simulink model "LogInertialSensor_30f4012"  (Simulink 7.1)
settings: Solver=FixedStepDiscrete  StartTime=0.0  StopTime=10.0  FixedStep=0.001  RelTol=1e-3
undefined symbols (not defined in the file or in its folder): bin2dec, bits, Buffer, characters, contain, empty, has, hex2dec, one, space, Transmit, When
libraries: dsPICdrivers x41, simulink x25

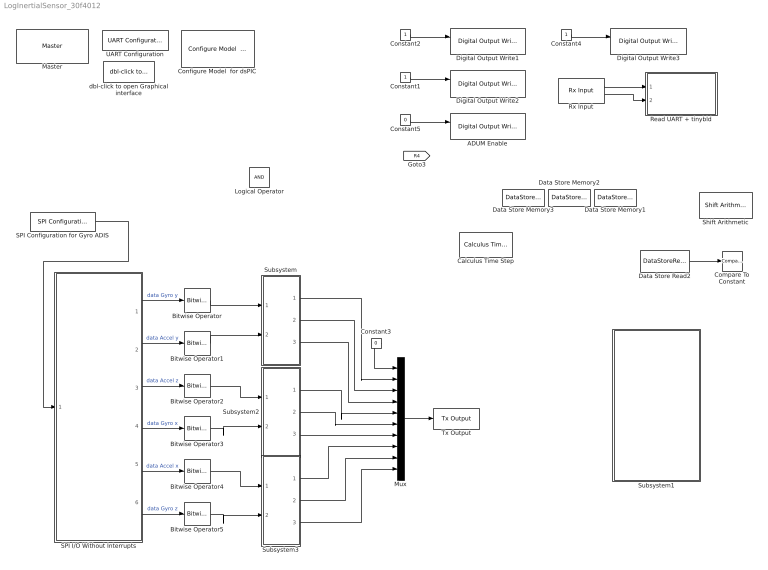
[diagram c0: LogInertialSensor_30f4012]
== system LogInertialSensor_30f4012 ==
  ADUM Enable : dsPICdrivers/Digital I//O/Digital Output Write  Tag=dsPIC_Digital_Output  Priority=5  PORT=E  Pin=1  Simultaneous=off  OrderingInOutPopup=Input
  Bitwise Operator{,1..5} (6 alike) : simulink/Logic and Bit Operations/Bitwise Operator  logicop=AND  UseBitMask=on  BitMask=hex2dec('0FFF')  BitMaskRealWorld=Stored Integer
  Calculus Time Step : dsPICdrivers/OTHERS/Calculus Time Step  Tag=dsPIC_CalculusTimeStep  SampleTime=.001  PR1chk=on
  Compare To Constant : simulink/Logic and Bit Operations/Compare To Constant  SystemSampleTime=-1  relop===  const=1  LogicOutDataTypeMode=uint8  ZeroCross=off
  Configure Model  for dsPIC : dsPICdrivers/Simulink Configuration/Configure Model  for dsPIC
  Constant1 : Constant  OutDataTypeMode=boolean  OutDataType=sfix(16)  OutScaling=2^0  OutDataTypeStr=boolean  SampleTime=-1
  Constant2 : Constant  OutDataTypeMode=boolean  OutDataType=sfix(16)  OutScaling=2^0  OutDataTypeStr=boolean  SampleTime=-1
  Constant3 : Constant  Value=0  OutDataTypeMode=uint8  OutDataType=sfix(16)  OutScaling=2^0  OutDataTypeStr=uint8  SampleTime=-1
  Constant4 : Constant  OutDataTypeMode=boolean  OutDataType=sfix(16)  OutScaling=2^0  OutDataTypeStr=boolean  SampleTime=-1
  Constant5 : Constant  Value=0  OutDataTypeMode=boolean  OutDataType=sfix(16)  OutScaling=2^0  OutDataTypeStr=boolean  SampleTime=-1
  Data Store Memory1 : DataStoreMemory  DataStoreName=Variable62  ReadBeforeWriteMsg=warning  WriteAfterWriteMsg=warning  WriteAfterReadMsg=warning  DataType=uint8  OutDataType=sfix(16)  OutScaling=2^0  OutDataTypeStr=uint8
  Data Store Memory2 : DataStoreMemory  DataStoreName=Variable61  ReadBeforeWriteMsg=warning  WriteAfterWriteMsg=warning  WriteAfterReadMsg=warning  DataType=uint8  OutDataType=sfix(16)  OutScaling=2^0  OutDataTypeStr=uint8
  Data Store Memory3 : DataStoreMemory  DataStoreName=Variable60  ReadBeforeWriteMsg=warning  WriteAfterWriteMsg=warning  WriteAfterReadMsg=warning  DataType=uint8  OutDataType=sfix(16)  OutScaling=2^0  OutDataTypeStr=uint8
  Data Store Read2 : DataStoreRead  DataStoreName=Variable60  SampleTime=.01
  Digital Output Write1 : dsPICdrivers/Digital I//O/Digital Output Write  Tag=dsPIC_Digital_Output  Priority=5  PORT=E  Pin=5  Simultaneous=off  OrderingInOutPopup=Input & Output
  Digital Output Write2 : dsPICdrivers/Digital I//O/Digital Output Write  Tag=dsPIC_Digital_Output  Priority=5  PORT=E  Pin=3  Simultaneous=off  OrderingInOutPopup=Input & Output
  Digital Output Write3 : dsPICdrivers/Digital I//O/Digital Output Write  Tag=dsPIC_Digital_Output  Priority=5  PORT=B  Pin=0  Simultaneous=off  OrderingInOutPopup=Input & Output
  Logical Operator : Logic  AllPortsSameDT=off  OutDataTypeMode=boolean  OutDataTypeStr=boolean
  Master : dsPICdrivers/Master  Tag=dsPIC_MASTER  Priority=1  TimeStepType=Timer1  picType=30f4012  fcy=20e6  Quartz_33f=5e6  PLLActive_33f=off  fcyDesired_33f=0  tmr1="[1  19999  0]"  tmr1Info="Time Step : 0.001  ;   Error : 0%  PR1=19999"  tmr2345="[0  0  0  0]"  tmr2345cfg=[-1 -1 -1 -1]  IOautoConf=on  typePort="[ 0   0   0   0   0   0   0   0   0   0   0   0   0   0   0   0  10   0   0   0   0   0   0   0   0   0   0   0   0   0   0   0   0   0   0   0   0   0   0   0   0   0   0   0   0   5   4   0   0   0   0   0   0   0   0   0   0   0   0   0   0   0   0   0   0  10   0  10   0  10   0   0  17   0   0   0   0   0   0   0   0   0  14  15   0   0   0   0   0   0   0   0   0   0   0   0   0   0   0   0 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"  TRIS="[ 65535  65534  65535  65535  65493  65535  65535 ]"  ADPCFG=1  MasterBusyPort=None  MasterOverloadPort=None  FOSC=XT_PLL8  ClockSwitchMonitor=Both disabled  TempProtection_33f=TEMP_ON  FPBOR=PBOR_OFF  PWRT=PWRT_4  MCLR=MCLR_DIS  PowerSave=off  OverrideFcy=off  NewFcy=1e6
  Mux : Mux  Inputs=10
  Read UART + tinybld : Subsystem  TreatAsAtomicUnit=on
  Rx Input : dsPICdrivers/Serial PORT/Rx Input  Tag=dsPIC_RX  Priority=5  UART=1  SampleTime=.01  BlockingFctChk=off  OutputDefault=0  IsPresentFlagChk=on
  SPI Configuration for Gyro ADIS : dsPICdrivers/SPI PORT/SPI Configuration  Tag=dsPIC_config_SPI  Priority=2  ConfigurationTime=At block execution (reconfigure on the fly)  OrderingInOutPopup=Output  SampleTime=-1  Frame_Enable=0  Frame_Sync=0  SPI=1  MODE=MASTER  USER_SCALER=2  StartEnable=Enable  SDO_EN=on  DATA_LENGTH=16 bits  SS_EN=off  SMP=Middle of bit  CKP=high  CKE=Idle to Active  Status="OK - Mode 1  -    Fsck= 10000000Hz"
  SPI I/O Without Interrupts : Subsystem
  Shift Arithmetic : simulink/Logic and Bit Operations/Shift Arithmetic  SystemSampleTime=-1  nBitShiftRight=8  nBinPtShiftRight=0
  Subsystem : Subsystem
  Subsystem1 : Subsystem
  Subsystem2 : Subsystem
  Subsystem3 : Subsystem
  Tx Output : dsPICdrivers/Serial PORT/Tx Output  Tag=dsPIC_TX  Priority=5  UART=1  OrderingInOutPopup=None
  UART Configuration : dsPICdrivers/Serial PORT/UART Configuration  Tag=dsPIC_config_UART  Priority=2  UART=1  proposed_BAUD=115200  ALT_TX_RX=on  InterruptTxWhen=When Transmit Buffer has one empty space (contain 3 characters)  TXInterruptPri=4  TxBufferSize=128  TXEN=on  InterruptRxWhen=When a character is received  RXInterruptPri=1  RxBufferSize=32  BAUD=115200  UxBRG=10  Info="UxBRG = 10   ||  Real Baud : 113636   ||  % error : -1.3573  ||  max 11.3636 Bytes / Step"  RealBaud=0
  dbl-click to open Graphical interface : dsPICdrivers/Serial PORT/dbl-click to open Graphical interface  SystemSampleTime=-1  Nothing=0
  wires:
  Constant2/1 -> Digital Output Write1/1
  Constant1/1 -> Digital Output Write2/1
  Constant5/1 -> ADUM Enable/1
  Rx Input/1 -> Read UART + tinybld/1(Rx)
  Rx Input/2 -> Read UART + tinybld/2(Flag)
  Constant4/1 -> Digital Output Write3/1
  SPI Configuration for Gyro ADIS/1 -> SPI I/O Without Interrupts/1(Ordering)
  SPI I/O Without Interrupts/1(Gyro y) -> Bitwise Operator/1  "data Gyro y"
  SPI I/O Without Interrupts/2(Accel y) -> Bitwise Operator1/1  "data Accel y"
  SPI I/O Without Interrupts/3(Accel z) -> Bitwise Operator2/1  "data Accel z"
  SPI I/O Without Interrupts/4(Gyro x) -> Bitwise Operator3/1  "data Gyro x"
  SPI I/O Without Interrupts/5(Accel x) -> Bitwise Operator4/1  "data Accel x"
  SPI I/O Without Interrupts/6(Gyro z) -> Bitwise Operator5/1  "data Gyro z"
  Data Store Read2/1 -> Compare To Constant/1
  Bitwise Operator/1 -> Subsystem/1(In1)
  Bitwise Operator1/1 -> Subsystem/2(In2)
  Bitwise Operator2/1 -> Subsystem2/1(In1)
  Bitwise Operator3/1 -> Subsystem2/2(In2)
  Bitwise Operator4/1 -> Subsystem3/1(In1)
  Bitwise Operator5/1 -> Subsystem3/2(In2)
  Mux/1 -> Tx Output/1
  Constant3/1 -> Mux/1
  Subsystem/1(Out1) -> Mux/2
  Subsystem/2(Out2) -> Mux/3
  Subsystem/3(Out3) -> Mux/4
  Subsystem2/1(Out1) -> Mux/5
  Subsystem2/2(Out2) -> Mux/6
  Subsystem2/3(Out3) -> Mux/7
  Subsystem3/1(Out1) -> Mux/8
  Subsystem3/2(Out2) -> Mux/9
  Subsystem3/3(Out3) -> Mux/10

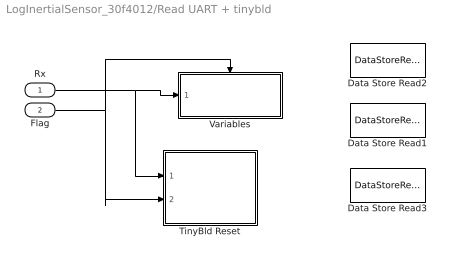
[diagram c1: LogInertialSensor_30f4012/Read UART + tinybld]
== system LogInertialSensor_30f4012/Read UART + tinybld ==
  Rx : Inport  OutDataType=sfix(16)  OutScaling=2^0
  Flag : Inport  Port=2  OutDataType=sfix(16)  OutScaling=2^0
  Data Store Read1 : DataStoreRead  DataStoreName=Variable61  SampleTime=.01
  Data Store Read2 : DataStoreRead  DataStoreName=Variable60  SampleTime=.01
  Data Store Read3 : DataStoreRead  DataStoreName=Variable62  SampleTime=.01
  TinyBld Reset : Subsystem  AncestorBlock=dsPICdrivers/OTHERS/TinyBld Reset
  Variables : Subsystem  TreatAsAtomicUnit=on
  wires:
  Flag/1 -> Variables/Enable, TinyBld Reset/2(Flag)
  Rx/1 -> Variables/1(In1), TinyBld Reset/1(Rx)

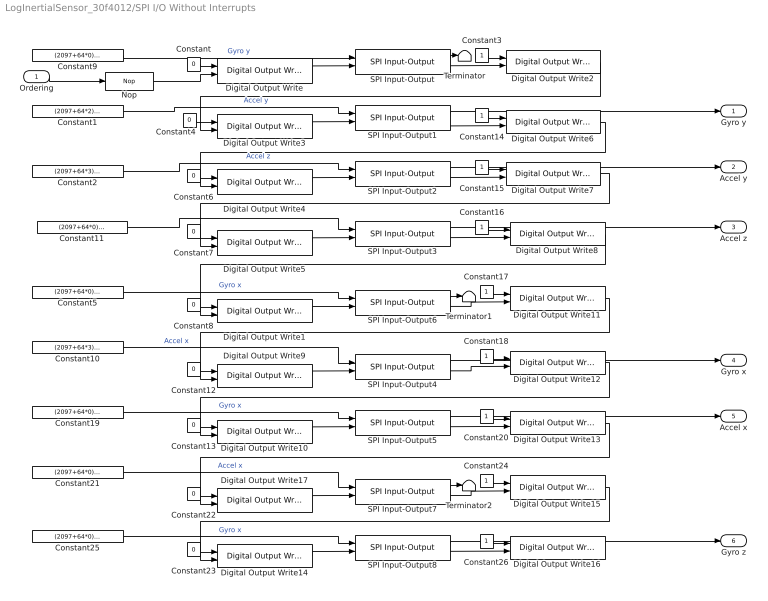
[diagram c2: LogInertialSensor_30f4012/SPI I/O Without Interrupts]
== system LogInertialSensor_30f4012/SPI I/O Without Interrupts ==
  Ordering : Inport  OutDataType=sfix(16)  OutScaling=2^0
  Constant{,4,6..8,12..13,22..23} (9 alike) : Constant  Value=0  OutDataTypeMode=boolean  OutDataType=sfix(16)  OutScaling=2^0  OutDataTypeStr=boolean
  Constant1 : Constant  Value=(2097+64*2)*16  VectorParams1D=off  OutDataTypeMode=uint16  OutDataType=sfix(16)  OutScaling=2^0  OutDataTypeStr=uint16  SampleTime=-1
  Constant10 : Constant  Value=(2097+64*3)*16  VectorParams1D=off  OutDataTypeMode=uint16  OutDataType=sfix(16)  OutScaling=2^0  OutDataTypeStr=uint16  SampleTime=-1
  Constant{5,9,11,19,21,25} (6 alike) : Constant  Value=(2097+64*0)*16  VectorParams1D=off  OutDataTypeMode=uint16  OutDataType=sfix(16)  OutScaling=2^0  OutDataTypeStr=uint16  SampleTime=-1
  Constant{3,14..18,20,24,26} (9 alike) : Constant  OutDataTypeMode=boolean  OutDataType=sfix(16)  OutScaling=2^0  OutDataTypeStr=boolean
  Constant2 : Constant  Value=(2097+64*3)*16  VectorParams1D=off  OutDataTypeMode=uint16  OutDataType=sfix(16)  OutScaling=2^0  OutDataTypeStr=uint16  SampleTime=-1
  Digital Output Write{,2..8} (8 alike) : dsPICdrivers/Digital I//O/Digital Output Write  Tag=dsPIC_Digital_Output  Priority=5  PORT=E  Pin=5  Simultaneous=off  OrderingInOutPopup=Input & Output
  Digital Output Write{1,9..13} (6 alike) : dsPICdrivers/Digital I//O/Digital Output Write  Tag=dsPIC_Digital_Output  Priority=5  PORT=E  Pin=3  Simultaneous=off  OrderingInOutPopup=Input & Output
  Digital Output Write14 : dsPICdrivers/Digital I//O/Digital Output Write  Tag=dsPIC_Digital_Output  Priority=5  PORT=B  Pin=0  Simultaneous=off  OrderingInOutPopup=Input & Output
  Digital Output Write15 : dsPICdrivers/Digital I//O/Digital Output Write  Tag=dsPIC_Digital_Output  Priority=5  PORT=B  Pin=0  Simultaneous=off  OrderingInOutPopup=Input & Output
  Digital Output Write16 : dsPICdrivers/Digital I//O/Digital Output Write  Tag=dsPIC_Digital_Output  Priority=5  PORT=B  Pin=0  Simultaneous=off  OrderingInOutPopup=Input
  Digital Output Write17 : dsPICdrivers/Digital I//O/Digital Output Write  Tag=dsPIC_Digital_Output  Priority=5  PORT=B  Pin=0  Simultaneous=off  OrderingInOutPopup=Input & Output
  Nop : dsPICdrivers/OTHERS/Nop  Tag=dsPIC_Reset  NbrNop=30
  SPI Input-Output{,1..8} (9 alike) : dsPICdrivers/SPI PORT/SPI Input-Output  Tag=dsPIC_SPI  SPI=1  INPUT=on  RESET_INPUT=off  OUTPUT=on  SPECIAL_SPI=Always Enable  DATA_LENGTH=16 bits  WAIT_INPUTDATA=on  OrderingInOutPopup=Input & Output  SampleTime=-1
  Terminator : Terminator
  Terminator1 : Terminator
  Terminator2 : Terminator
  Gyro y : Outport
  Accel y : Outport  Port=2
  Accel z : Outport  Port=3
  Gyro x : Outport  Port=4
  Accel x : Outport  Port=5
  Gyro z : Outport  Port=6
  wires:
  SPI Input-Output7/1 -> Terminator2/1
  Constant25/1 -> SPI Input-Output8/1  "Gyro x"
  Constant21/1 -> SPI Input-Output7/1  "Accel x"
  Constant22/1 -> Digital Output Write17/1
  Constant23/1 -> Digital Output Write14/1
  Digital Output Write17/1 -> SPI Input-Output7/2
  Digital Output Write14/1 -> SPI Input-Output8/2
  Constant24/1 -> Digital Output Write15/1
  Constant26/1 -> Digital Output Write16/1
  SPI Input-Output7/2 -> Digital Output Write15/2
  SPI Input-Output8/2 -> Digital Output Write16/2
  Digital Output Write13/1 -> Digital Output Write17/2
  Digital Output Write15/1 -> Digital Output Write14/2
  SPI Input-Output8/1 -> Gyro z/1
  Nop/1 -> Digital Output Write/2
  Ordering/1 -> Nop/1
  Constant19/1 -> SPI Input-Output5/1  "Gyro x"
  Constant10/1 -> SPI Input-Output4/1  "Accel x"
  Constant5/1 -> SPI Input-Output6/1  "Gyro x"
  Constant11/1 -> SPI Input-Output3/1
  Constant2/1 -> SPI Input-Output2/1  "Accel z"
  Constant1/1 -> SPI Input-Output1/1  "Accel y"
  Constant9/1 -> SPI Input-Output/1  "Gyro y"
  Constant/1 -> Digital Output Write/1
  Constant3/1 -> Digital Output Write2/1
  SPI Input-Output/2 -> Digital Output Write2/2
  Digital Output Write/1 -> SPI Input-Output/2
  Constant6/1 -> Digital Output Write4/1
  Digital Output Write4/1 -> SPI Input-Output2/2
  Constant7/1 -> Digital Output Write5/1
  Digital Output Write5/1 -> SPI Input-Output3/2
  Constant4/1 -> Digital Output Write3/1
  Digital Output Write3/1 -> SPI Input-Output1/2
  Digital Output Write2/1 -> Digital Output Write3/2
  Constant14/1 -> Digital Output Write6/1
  SPI Input-Output1/2 -> Digital Output Write6/2
  Constant15/1 -> Digital Output Write7/1
  Constant16/1 -> Digital Output Write8/1
  SPI Input-Output2/2 -> Digital Output Write7/2
  SPI Input-Output3/2 -> Digital Output Write8/2
  Digital Output Write6/1 -> Digital Output Write4/2
  Digital Output Write7/1 -> Digital Output Write5/2
  Constant8/1 -> Digital Output Write1/1
  Constant12/1 -> Digital Output Write9/1
  Constant13/1 -> Digital Output Write10/1
  Digital Output Write1/1 -> SPI Input-Output6/2
  Digital Output Write9/1 -> SPI Input-Output4/2
  Digital Output Write10/1 -> SPI Input-Output5/2
  Digital Output Write8/1 -> Digital Output Write1/2
  Constant17/1 -> Digital Output Write11/1
  Constant18/1 -> Digital Output Write12/1
  Constant20/1 -> Digital Output Write13/1
  SPI Input-Output6/2 -> Digital Output Write11/2
  SPI Input-Output4/2 -> Digital Output Write12/2
  SPI Input-Output5/2 -> Digital Output Write13/2
  Digital Output Write11/1 -> Digital Output Write9/2
  Digital Output Write12/1 -> Digital Output Write10/2
  SPI Input-Output1/1 -> Gyro y/1
  SPI Input-Output2/1 -> Accel y/1
  SPI Input-Output3/1 -> Accel z/1
  SPI Input-Output4/1 -> Gyro x/1
  SPI Input-Output5/1 -> Accel x/1
  SPI Input-Output/1 -> Terminator/1
  SPI Input-Output6/1 -> Terminator1/1

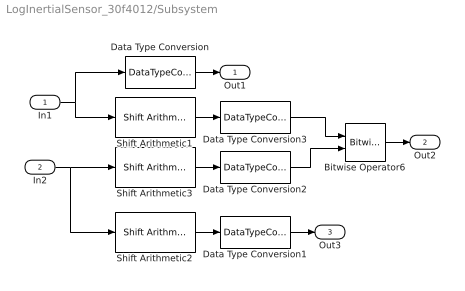
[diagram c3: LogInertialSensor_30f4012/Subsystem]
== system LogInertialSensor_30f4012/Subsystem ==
  In1 : Inport
  In2 : Inport  Port=2
  Bitwise Operator6 : simulink/Logic and Bit Operations/Bitwise Operator  logicop=OR  UseBitMask=off  NumInputPorts=2  BitMask=bin2dec('11011001')  BitMaskRealWorld=Stored Integer
  Data Type Conversion{,1..3} (4 alike) : DataTypeConversion  OutDataTypeMode=uint8  OutDataType=sfix(16)  OutScaling=2^0  OutDataTypeStr=uint8  ConvertRealWorld=Stored Integer (SI)
  Shift Arithmetic1 : simulink/Logic and Bit Operations/Shift Arithmetic  SystemSampleTime=-1  nBitShiftRight=8  nBinPtShiftRight=0
  Shift Arithmetic2 : simulink/Logic and Bit Operations/Shift Arithmetic  SystemSampleTime=-1  nBitShiftRight=4  nBinPtShiftRight=0
  Shift Arithmetic3 : simulink/Logic and Bit Operations/Shift Arithmetic  SystemSampleTime=-1  nBitShiftRight=-4  nBinPtShiftRight=0
  Out1 : Outport
  Out2 : Outport  Port=2
  Out3 : Outport  Port=3
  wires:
  In1/1 -> Shift Arithmetic1/1, Data Type Conversion/1
  In2/1 -> Shift Arithmetic3/1, Shift Arithmetic2/1
  Shift Arithmetic2/1 -> Data Type Conversion1/1
  Shift Arithmetic3/1 -> Data Type Conversion2/1
  Data Type Conversion2/1 -> Bitwise Operator6/2
  Shift Arithmetic1/1 -> Data Type Conversion3/1
  Data Type Conversion/1 -> Out1/1
  Bitwise Operator6/1 -> Out2/1
  Data Type Conversion1/1 -> Out3/1
  Data Type Conversion3/1 -> Bitwise Operator6/1

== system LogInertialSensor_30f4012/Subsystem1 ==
  Enable : EnablePort  StatesWhenEnabling=reset

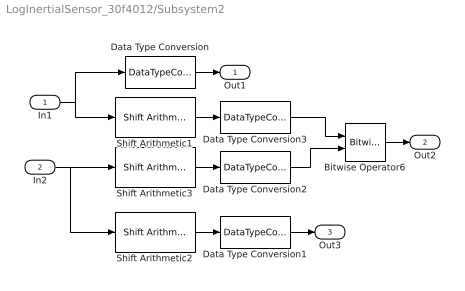
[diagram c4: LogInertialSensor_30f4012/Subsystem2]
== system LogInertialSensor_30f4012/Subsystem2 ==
  In1 : Inport
  In2 : Inport  Port=2
  Bitwise Operator6 : simulink/Logic and Bit Operations/Bitwise Operator  logicop=OR  UseBitMask=off  NumInputPorts=2  BitMask=bin2dec('11011001')  BitMaskRealWorld=Stored Integer
  Data Type Conversion{,1..3} (4 alike) : DataTypeConversion  OutDataTypeMode=uint8  OutDataType=sfix(16)  OutScaling=2^0  OutDataTypeStr=uint8  ConvertRealWorld=Stored Integer (SI)
  Shift Arithmetic1 : simulink/Logic and Bit Operations/Shift Arithmetic  SystemSampleTime=-1  nBitShiftRight=8  nBinPtShiftRight=0
  Shift Arithmetic2 : simulink/Logic and Bit Operations/Shift Arithmetic  SystemSampleTime=-1  nBitShiftRight=4  nBinPtShiftRight=0
  Shift Arithmetic3 : simulink/Logic and Bit Operations/Shift Arithmetic  SystemSampleTime=-1  nBitShiftRight=-4  nBinPtShiftRight=0
  Out1 : Outport
  Out2 : Outport  Port=2
  Out3 : Outport  Port=3
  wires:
  Data Type Conversion3/1 -> Bitwise Operator6/1
  Data Type Conversion1/1 -> Out3/1
  Bitwise Operator6/1 -> Out2/1
  Data Type Conversion/1 -> Out1/1
  Shift Arithmetic1/1 -> Data Type Conversion3/1
  Data Type Conversion2/1 -> Bitwise Operator6/2
  Shift Arithmetic3/1 -> Data Type Conversion2/1
  Shift Arithmetic2/1 -> Data Type Conversion1/1
  In2/1 -> Shift Arithmetic2/1, Shift Arithmetic3/1
  In1/1 -> Data Type Conversion/1, Shift Arithmetic1/1

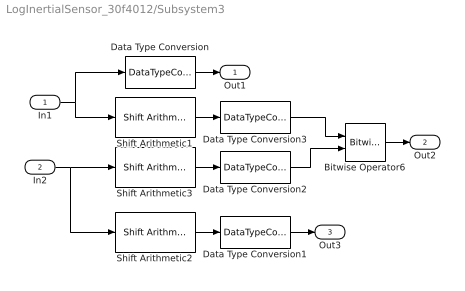
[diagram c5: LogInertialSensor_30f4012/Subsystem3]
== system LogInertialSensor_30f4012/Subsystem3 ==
  In1 : Inport
  In2 : Inport  Port=2
  Bitwise Operator6 : simulink/Logic and Bit Operations/Bitwise Operator  logicop=OR  UseBitMask=off  NumInputPorts=2  BitMask=bin2dec('11011001')  BitMaskRealWorld=Stored Integer
  Data Type Conversion{,1..3} (4 alike) : DataTypeConversion  OutDataTypeMode=uint8  OutDataType=sfix(16)  OutScaling=2^0  OutDataTypeStr=uint8  ConvertRealWorld=Stored Integer (SI)
  Shift Arithmetic1 : simulink/Logic and Bit Operations/Shift Arithmetic  SystemSampleTime=-1  nBitShiftRight=8  nBinPtShiftRight=0
  Shift Arithmetic2 : simulink/Logic and Bit Operations/Shift Arithmetic  SystemSampleTime=-1  nBitShiftRight=4  nBinPtShiftRight=0
  Shift Arithmetic3 : simulink/Logic and Bit Operations/Shift Arithmetic  SystemSampleTime=-1  nBitShiftRight=-4  nBinPtShiftRight=0
  Out1 : Outport
  Out2 : Outport  Port=2
  Out3 : Outport  Port=3
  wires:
  In1/1 -> Shift Arithmetic1/1, Data Type Conversion/1
  In2/1 -> Shift Arithmetic3/1, Shift Arithmetic2/1
  Shift Arithmetic2/1 -> Data Type Conversion1/1
  Shift Arithmetic3/1 -> Data Type Conversion2/1
  Data Type Conversion2/1 -> Bitwise Operator6/2
  Shift Arithmetic1/1 -> Data Type Conversion3/1
  Data Type Conversion/1 -> Out1/1
  Bitwise Operator6/1 -> Out2/1
  Data Type Conversion1/1 -> Out3/1
  Data Type Conversion3/1 -> Bitwise Operator6/1

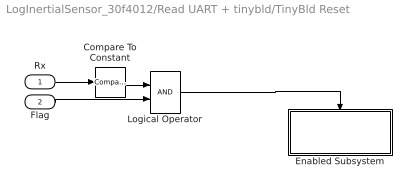
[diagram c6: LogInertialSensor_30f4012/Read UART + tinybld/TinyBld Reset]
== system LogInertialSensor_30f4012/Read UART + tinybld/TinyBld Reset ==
  Rx : Inport  OutDataType=sfix(16)  OutScaling=2^0
  Flag : Inport  Port=2  OutDataType=sfix(16)  OutScaling=2^0
  Compare To Constant : simulink/Logic and Bit Operations/Compare To Constant  SystemSampleTime=-1  relop===  const=55  LogicOutDataTypeMode=boolean  ZeroCross=off
  Enabled Subsystem : Subsystem  TreatAsAtomicUnit=on
  Logical Operator : Logic  AllPortsSameDT=off  OutDataTypeMode=boolean  OutDataTypeStr=boolean
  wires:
  Rx/1 -> Compare To Constant/1
  Compare To Constant/1 -> Logical Operator/1
  Flag/1 -> Logical Operator/2
  Logical Operator/1 -> Enabled Subsystem/Enable

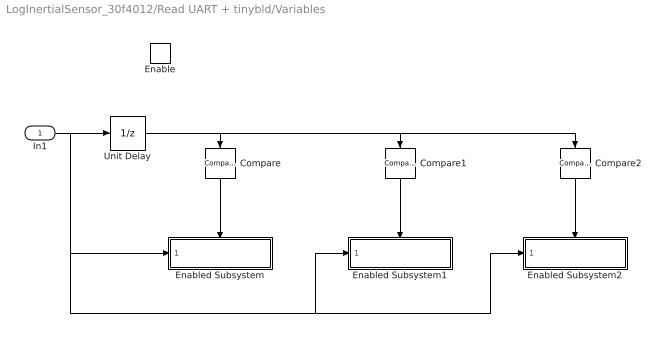
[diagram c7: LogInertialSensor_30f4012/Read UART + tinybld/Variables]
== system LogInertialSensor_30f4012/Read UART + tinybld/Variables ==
  In1 : Inport  OutDataType=sfix(16)  OutScaling=2^0
  Enable : EnablePort
  Compare : simulink/Logic and Bit Operations/Compare To Constant  Orientation=down  SystemSampleTime=-1  relop===  const=60  LogicOutDataTypeMode=boolean  ZeroCross=off
  Compare1 : simulink/Logic and Bit Operations/Compare To Constant  Orientation=down  SystemSampleTime=-1  relop===  const=61  LogicOutDataTypeMode=boolean  ZeroCross=off
  Compare2 : simulink/Logic and Bit Operations/Compare To Constant  Orientation=down  SystemSampleTime=-1  relop===  const=61  LogicOutDataTypeMode=boolean  ZeroCross=off
  Enabled Subsystem : Subsystem  TreatAsAtomicUnit=on
  Enabled Subsystem1 : Subsystem  TreatAsAtomicUnit=on
  Enabled Subsystem2 : Subsystem  TreatAsAtomicUnit=on
  Unit Delay : UnitDelay  SampleTime=-1
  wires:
  Compare2/1 -> Enabled Subsystem2/Enable
  In1/1 -> Unit Delay/1, Enabled Subsystem2/1(In1), Enabled Subsystem1/1(In1), Enabled Subsystem/1(In1)
  Unit Delay/1 -> Compare2/1, Compare1/1, Compare/1
  Compare/1 -> Enabled Subsystem/Enable
  Compare1/1 -> Enabled Subsystem1/Enable

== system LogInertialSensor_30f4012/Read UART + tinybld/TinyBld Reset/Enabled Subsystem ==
  Enable : EnablePort
  While Iterator Subsystem : Subsystem  TreatAsAtomicUnit=on

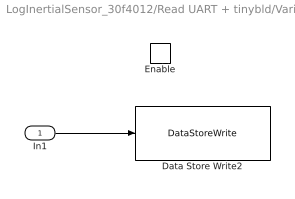
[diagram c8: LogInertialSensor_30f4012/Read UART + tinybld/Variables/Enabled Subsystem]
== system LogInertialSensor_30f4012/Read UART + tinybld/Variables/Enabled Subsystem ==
  In1 : Inport  OutDataType=sfix(16)  OutScaling=2^0
  Enable : EnablePort
  Data Store Write2 : DataStoreWrite  DataStoreName=Variable60  SampleTime=-1
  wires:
  In1/1 -> Data Store Write2/1

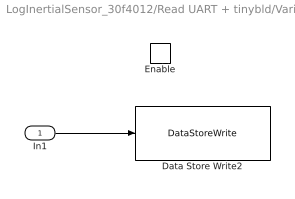
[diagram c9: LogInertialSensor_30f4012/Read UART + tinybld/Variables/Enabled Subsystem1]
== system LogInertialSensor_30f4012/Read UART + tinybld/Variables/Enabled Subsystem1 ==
  In1 : Inport  OutDataType=sfix(16)  OutScaling=2^0
  Enable : EnablePort
  Data Store Write2 : DataStoreWrite  DataStoreName=Variable61  SampleTime=-1
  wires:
  In1/1 -> Data Store Write2/1

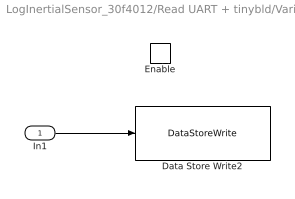
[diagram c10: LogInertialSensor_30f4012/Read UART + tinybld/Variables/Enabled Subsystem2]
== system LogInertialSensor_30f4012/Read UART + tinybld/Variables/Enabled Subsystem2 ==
  In1 : Inport  OutDataType=sfix(16)  OutScaling=2^0
  Enable : EnablePort
  Data Store Write2 : DataStoreWrite  DataStoreName=Variable62  SampleTime=-1
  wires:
  In1/1 -> Data Store Write2/1

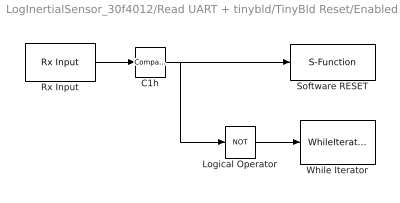
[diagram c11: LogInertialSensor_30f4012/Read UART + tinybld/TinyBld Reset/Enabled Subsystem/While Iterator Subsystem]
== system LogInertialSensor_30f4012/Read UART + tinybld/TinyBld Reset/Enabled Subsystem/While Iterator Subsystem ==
  C1h : simulink/Logic and Bit Operations/Compare To Constant  SystemSampleTime=-1  relop===  const=66  LogicOutDataTypeMode=boolean  ZeroCross=off
  Logical Operator : Logic  Operator=NOT  AllPortsSameDT=off  OutDataTypeMode=boolean  OutDataTypeStr=boolean
  Rx Input : dsPICdrivers/Serial PORT/Rx Input  Tag=dsPIC_RX  Priority=5  UART=1  SampleTime=-1  BlockingFctChk=on  OutputDefault=0  IsPresentFlagChk=off
  Software RESET : S-Function  Tag=dsPIC_Reset  FunctionName=dsPIC_Reset  EnableBusSupport=off
  While Iterator : WhileIterator  MaxIters=-1  WhileBlockType=do-while  ResetStates=reset
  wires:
  Logical Operator/1 -> While Iterator/1
  Rx Input/1 -> C1h/1
  C1h/1 -> Software RESET/1, Logical Operator/1
